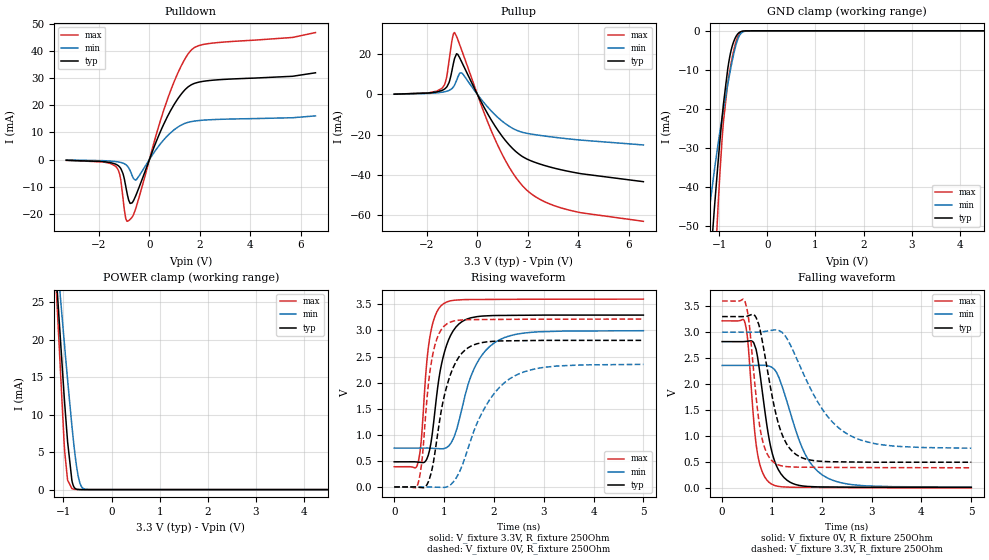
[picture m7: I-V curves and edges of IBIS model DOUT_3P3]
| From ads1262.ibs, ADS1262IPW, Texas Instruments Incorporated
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|   Model DOUT_3P3
[Model]   DOUT_3P3
Model_type   3-state
Polarity   Non-Inverting
Enable   Active-Low
Vmeas = 1.65
Vref = 3.3
Cref = 15pF
Rref = 250
|   typ   min   max
|   (nom PVT)   (Fast PVT)   (slow PVT)
|   (nom PVT)   (slow PVT)   (fast PVT)
C_comp   0.294p   0.276p   0.334p
|C_comp (ON state)   0.308p   0.292p   0.350p
|C_comp (OFF state)   0.294p   0.276p   0.334p
| Where   nom PVT is  Nominal Process, 3.3V, 27C
|   Fast PVT is Strong Process, 3.6V, -40C
|   Slow PVT is Weak Process, 3.0V, 125C
[Voltage Range]   3.3   3.0   3.6
[Temperature Range]   27   125   -40
[Pullup Reference]   3.3   3.0   3.6
[Pulldown Reference]   0   0   0
[Power Clamp Reference]   3.3   3.0   3.6
[GND Clamp Reference]   0   0   0
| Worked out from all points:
|   slope of the pulldown table from 0 to 0.495 V, typ, clamps not added: 42.9 ohm
|   slope of the pullup table from 0 to 0.495 V, typ, clamps not added: 42.9 ohm
|   GND clamp passes 1 mA (typ) near -0.63 V on its own axis
|   POWER clamp passes 1 mA (typ) near -0.82 V on its own axis
|   falling waveform, V_fixture 0V, R_fixture 250Ohm: 20-80 % time 284ps typ, 543ps min, 176ps max; typ from 2.82 V to 0.011 V
|   rising waveform, V_fixture 3.3V, R_fixture 250Ohm: 20-80 % time 289ps typ, 496ps min, 177ps max; typ from 0.482 V to 3.29 V
|   rising waveform, V_fixture 0V, R_fixture 250Ohm: 20-80 % time 365ps typ, 699ps min, 210ps max; typ from 0 V to 2.81 V
|   falling waveform, V_fixture 3.3V, R_fixture 250Ohm: 20-80 % time 370ps typ, 809ps min, 218ps max; typ from 3.3 V to 0.495 V
[Pulldown]
|   Voltage   I(typ)   I(min)   I(max)
-3.3V     -288.8uA   -187.2uA   -310.5uA
-1.34V    -1.715mA   -753.8uA   -2.528mA
-1.181V   -2.776mA   -994.6uA   -5.449mA
-1.053V   -5.12mA    -1.335mA   -13.96mA
-933.9mV  -10.15mA   -1.922mA   -21.94mA
-825mV    -14.96mA   -3.027mA   -22.58mA
-686.4mV  -15.99mA   -5.901mA   -21.29mA
-528mV    -13.03mA   -7.485mA   -17.65mA
699.6mV   15.57mA    8.594mA    21.81mA
1.254V    24.04mA    12.67mA    34.4mA
1.67V     27.63mA    14.01mA    40.51mA
6.59V     32.02mA    16.11mA    46.86mA
[GND Clamp]
|   Voltage   I(typ)   I(min)   I(max)
-3.3V     -480.5mA   -312.5mA   -681.8mA
-1.251V   -70.36mA   -50.02mA   -102.2mA
-1.102V   -45.49mA   -35.7mA    -63.47mA
-1.092V   -43.91mA   -34.8mA    -60.99mA
-1.023V   -33.33mA   -28.74mA   -44.38mA
-983.4mV  -27.67mA   -25.51mA   -35.72mA
-914.1mV  -18.78mA   -20.24mA   -23.35mA
-825mV    -9.842mA   -13.85mA   -13.48mA
-706.2mV  -2.973mA   -6.253mA   -5.381mA
-627mV    -969.5uA   -2.576mA   -1.836mA
-547.8mV  -195.7uA   -644.4uA   -323.8uA
6.59V     0A         0A         0A
[Pullup]
|   Voltage   I(typ)   I(min)   I(max)
-3.3V     53.73uA    56.19uA    35.81uA
-1.389V   1.99mA     1.033mA    3.193mA
-1.221V   3.545mA    1.486mA    8.315mA
-1.122V   5.872mA    1.939mA    16.66mA
-993.3mV  12.67mA    3.034mA    27.68mA
-904.2mV  17.8mA     4.568mA    30.64mA
-825mV    20.13mA    6.844mA    28.77mA
-617.1mV  15.96mA    10.59mA    21.76mA
798.6mV   -17.59mA   -11.33mA   -25.04mA
1.947V    -32.04mA   -19.35mA   -47.43mA
3.472V    -37.91mA   -21.95mA   -56.97mA
6.59V     -43.42mA   -25.17mA   -63.11mA
[POWER Clamp]
|   Voltage   I(typ)   I(min)   I(max)
-3.3V     137.8mA    122.6mA    153.3mA
-1.439V   56.85mA    53.71mA    63.2mA
-983.4mV  12.33mA    19.75mA    5.968mA
-973.5mV  11.44mA    19.02mA    5.05mA
-914.1mV  6.424mA    14.68mA    1.272mA
-825mV    1.262mA    8.582mA    146.7uA
-815.1mV  966.7uA    7.951mA    118.2uA
-745.8mV  111.1uA    3.995mA    22.11uA
-686.4mV  16.8uA     1.593mA    4.149uA
-627mV    2.833uA    423.4uA    628.5nA
-537.9mV  179.2nA    37.61uA    9.442nA
6.59V     0A         0A         0A
[Ramp]
R_load = 250
|   typ   min   max
dV/dt_r   1.68714/2.89388e-10   1.34966/4.96069e-10   1.9276/1.77036e-10
dV/dt_f   1.6839/2.83654e-10   1.40634/5.42729e-10   1.93006/1.75858e-10
[Falling Waveform]
V_fixture = 0V
V_fixture_min = 0V
V_fixture_max = 0V
R_fixture = 250Ohm
C_fixture = 0F
|   Time   V(typ)   V(min)   V(max)
0s        2.818V     2.358V     3.218V
461.7ps   2.82V      2.36V      3.17V
513.1ps   2.826V     2.36V      2.856V
643.4ps   2.772V     2.36V      1.191V
706.2ps   2.548V     2.36V      681.8mV
989.6ps   730.8mV    2.326V     74.35mV
1.3ns     149.7mV    1.667V     16.54mV
1.652ns   33.58mV    675.4mV    10.61mV
2.02ns    18.62mV    243.2mV    8.555mV
5ns       11.19mV    14.35mV    884uV
[Rising Waveform]
V_fixture = 3.3V
V_fixture_min = 3V
V_fixture_max = 3.6V
R_fixture = 250Ohm
C_fixture = 0F
|   Time   V(typ)   V(min)   V(max)
0s        481.6mV    744.8mV    387mV
478.8ps   475.8mV    745mV      466mV
547.5ps   469.1mV    745mV      942.3mV
643.4ps   516.6mV    745mV      2.281V
706.2ps   690.7mV    743.6mV    2.818V
989.6ps   2.516V     734.3mV    3.512V
1.3ns     3.125V     1.267V     3.585V
1.596ns   3.252V     2.251V     3.592V
2.02ns    3.286V     2.769V     3.594V
5ns       3.293V     2.994V     3.6V
[Rising Waveform]
V_fixture = 0V
V_fixture_min = 0V
V_fixture_max = 0V
R_fixture = 250Ohm
C_fixture = 0F
|   Time   V(typ)   V(min)   V(max)
0s        1.327nV    2.966nV    1.089nV
478.8ps   -4.748mV   179.5uV    67.93mV
564.6ps   -13.37mV   211.7uV    571.4mV
661.7ps   51.93mV    248.1uV    1.732V
755.3ps   325mV      -1.076mV   2.446V
1.053ns   1.924V     -89.92uV   3.124V
1.48ns    2.665V     733.6mV    3.206V
1.835ns   2.778V     1.548V     3.209V
2.32ns    2.801V     2.074V     3.212V
5ns       2.809V     2.349V     3.217V
[Falling Waveform]
|Gnd
V_fixture = 3.3V
V_fixture_min = 3V
V_fixture_max = 3.6V
R_fixture = 250Ohm
C_fixture = 0F
|   Time   V(typ)   V(min)   V(max)
0s        3.3V       3V         3.6V
461.7ps   3.302V     3V         3.584V
547.5ps   3.323V     3V         3.137V
782.2ps   2.95V      3.005V     1.035V
1.053ns   1.535V     3.044V     479.5mV
1.24ns    945.4mV    2.96V      417.3mV
1.48ns    645.8mV    2.525V     400.7mV
2.02ns    511mV      1.502V     396.3mV
2.52ns    500.1mV    1.034V     393.1mV
5ns       494.6mV    764.5mV    387.8mV
